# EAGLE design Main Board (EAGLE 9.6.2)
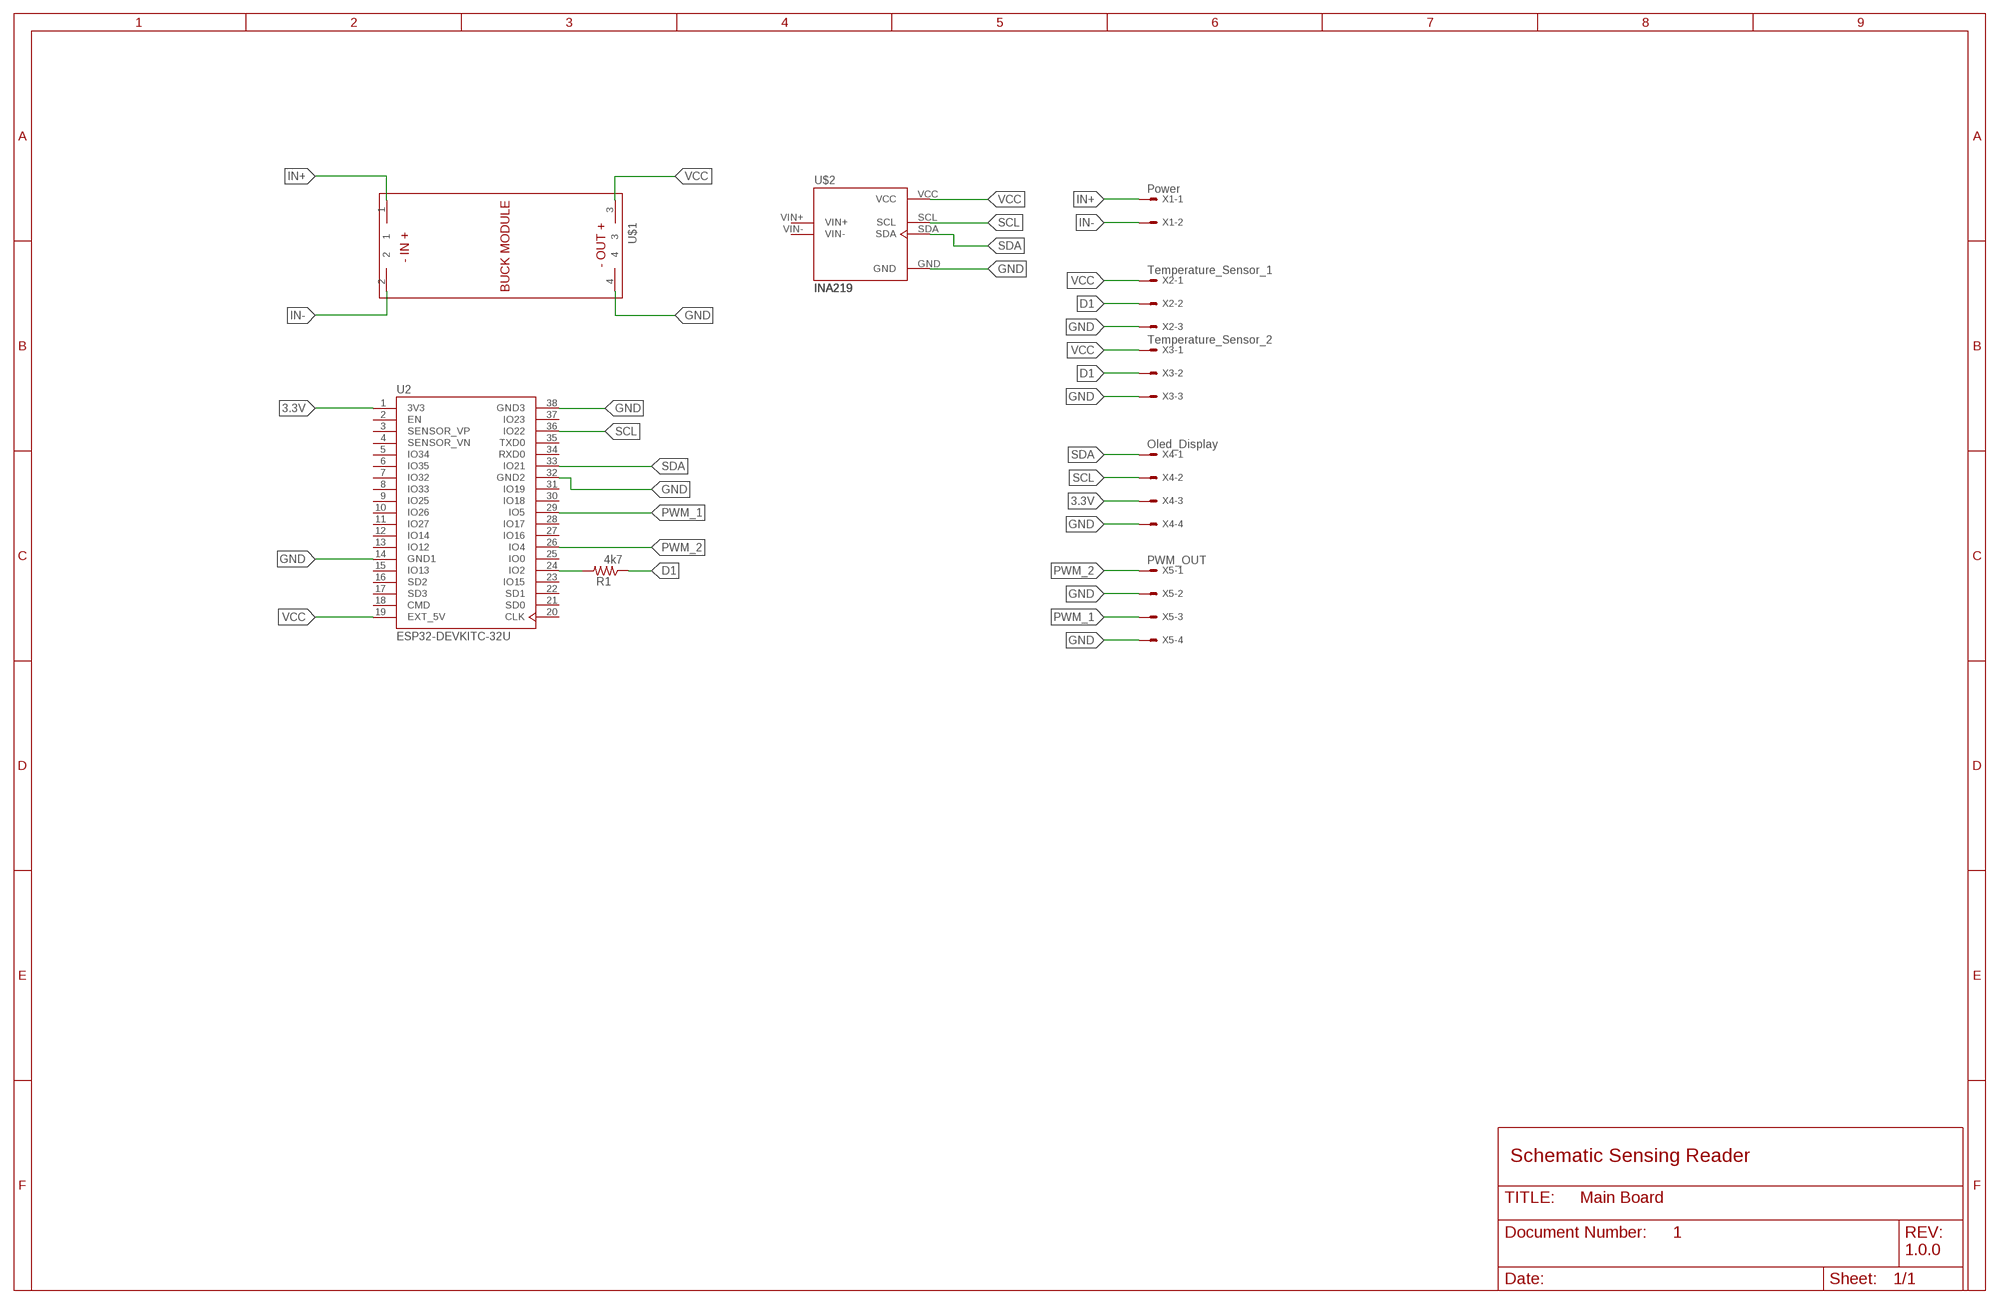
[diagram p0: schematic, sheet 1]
FRAME1 (FRAME_B_L): DESIGNER: PRATIK MAKWANA; DOC: 1; REV: 1.0.0

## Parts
R1  4k7  R-US_0207/10  [0207/10]
U2  ESP32-DEVKITC-32U  [MODULE_ESP32-DEVKITC-32U]
U$1  BUCK_MODULEWITH_SMDPADS&THROUGHHOLES  [BUCK_MODULE]
U$2  INA219  [INA219]
X1  Power  22-23-2021  [22-23-2021]
X2  Temperature_Sensor_1  22-23-2031  [22-23-2031]
X3  Temperature_Sensor_2  22-23-2031  [22-23-2031]
X4  Oled_Display  22-23-2041  [22-23-2041]
X5  PWM_OUT  22-23-2041  [22-23-2041]

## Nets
3.3V: U2.1(3V3) X4.3
D1: R1.1 X2.2 X3.2
GND: U2.14(GND1) U2.32(GND2) U2.38(GND3) U$1.4 U$2.GND X2.3 X3.3 X4.4 X5.2 X5.4
IN+: U$1.1 X1.1
IN-: U$1.2 X1.2
N$1: R1.2 U2.24(IO2)
PWM_1: U2.29(IO5) X5.3
PWM_2: U2.26(IO4) X5.1
SCL: U2.36(IO22) U$2.SCL X4.2
SDA: U2.33(IO21) U$2.SDA X4.1
VCC: U2.19(EXT_5V) U$1.3 U$2.VCC X2.1 X3.1
Unconnected: U2.2(EN) U2.3(SENSOR_VP) U2.4(SENSOR_VN) U2.5(IO34) U2.6(IO35) U2.7(IO32) U2.8(IO33) U2.9(IO25) U2.10(IO26) U2.11(IO27) U2.12(IO14) U2.13(IO12) U2.15(IO13) U2.16(SD2) U2.17(SD3) U2.18(CMD) U2.20(CLK) U2.21(SD0) U2.22(SD1) U2.23(IO15) U2.25(IO0) U2.27(IO16) U2.28(IO17) U2.30(IO18) U2.31(IO19) U2.34(RXD0) U2.35(TXD0) U2.37(IO23) U$2.VIN+ U$2.VIN-

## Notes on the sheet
- Schematic Sensing Reader

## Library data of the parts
R1 = adafruit:R-US_: RESISTOR, American symbol
U2 = ESP32-DEVKITC-32U:ESP32-DEVKITC-32U: Check availability; AVAILABILITY: In Stock; CHECK_PRICES: https://www.snapeda.com/parts/ESP32-DEVKITC-32U/Espressif+Systems/view-part/?ref=eda; DESCRIPTION: ESP32-WROOM-32UE series Transceiver; 802.11 b/g/n (Wi-Fi, WiFi, WLAN), Bluetooth® Smart Ready 4.x Dual Mode Evaluation Board; MF: Espressif Systems; MP: ESP32-DEVKITC-32U; PACKAGE: CUSTOM-38 ESPRESSIF; PRICE: None; SNAPEDA_LINK: https://www.snapeda.com/parts/ESP32-DEVKITC-32U/Espressif+Systems/view-part/?ref=snap
U$1 = BUCK_MODULE:BUCK_MODULE
U$2 = INA219:INA219
X1 = con-molex:22-23-2021: .100" (2.54mm) Center Header - 2 Pin; MF: MOLEX; MPN: 22-23-2021; OC_FARNELL: 1462926; OC_NEWARK: 25C3832
X2 X3 = con-molex:22-23-2031: .100" (2.54mm) Center Header - 3 Pin; MF: MOLEX; MPN: 22-23-2031; OC_FARNELL: 1462950; OC_NEWARK: 30C0862
X4 X5 = con-molex:22-23-2041: .100" (2.54mm) Center Header - 4 Pin; MF: MOLEX; MPN: 22-23-2041; OC_FARNELL: 1462920; OC_NEWARK: 38C0355

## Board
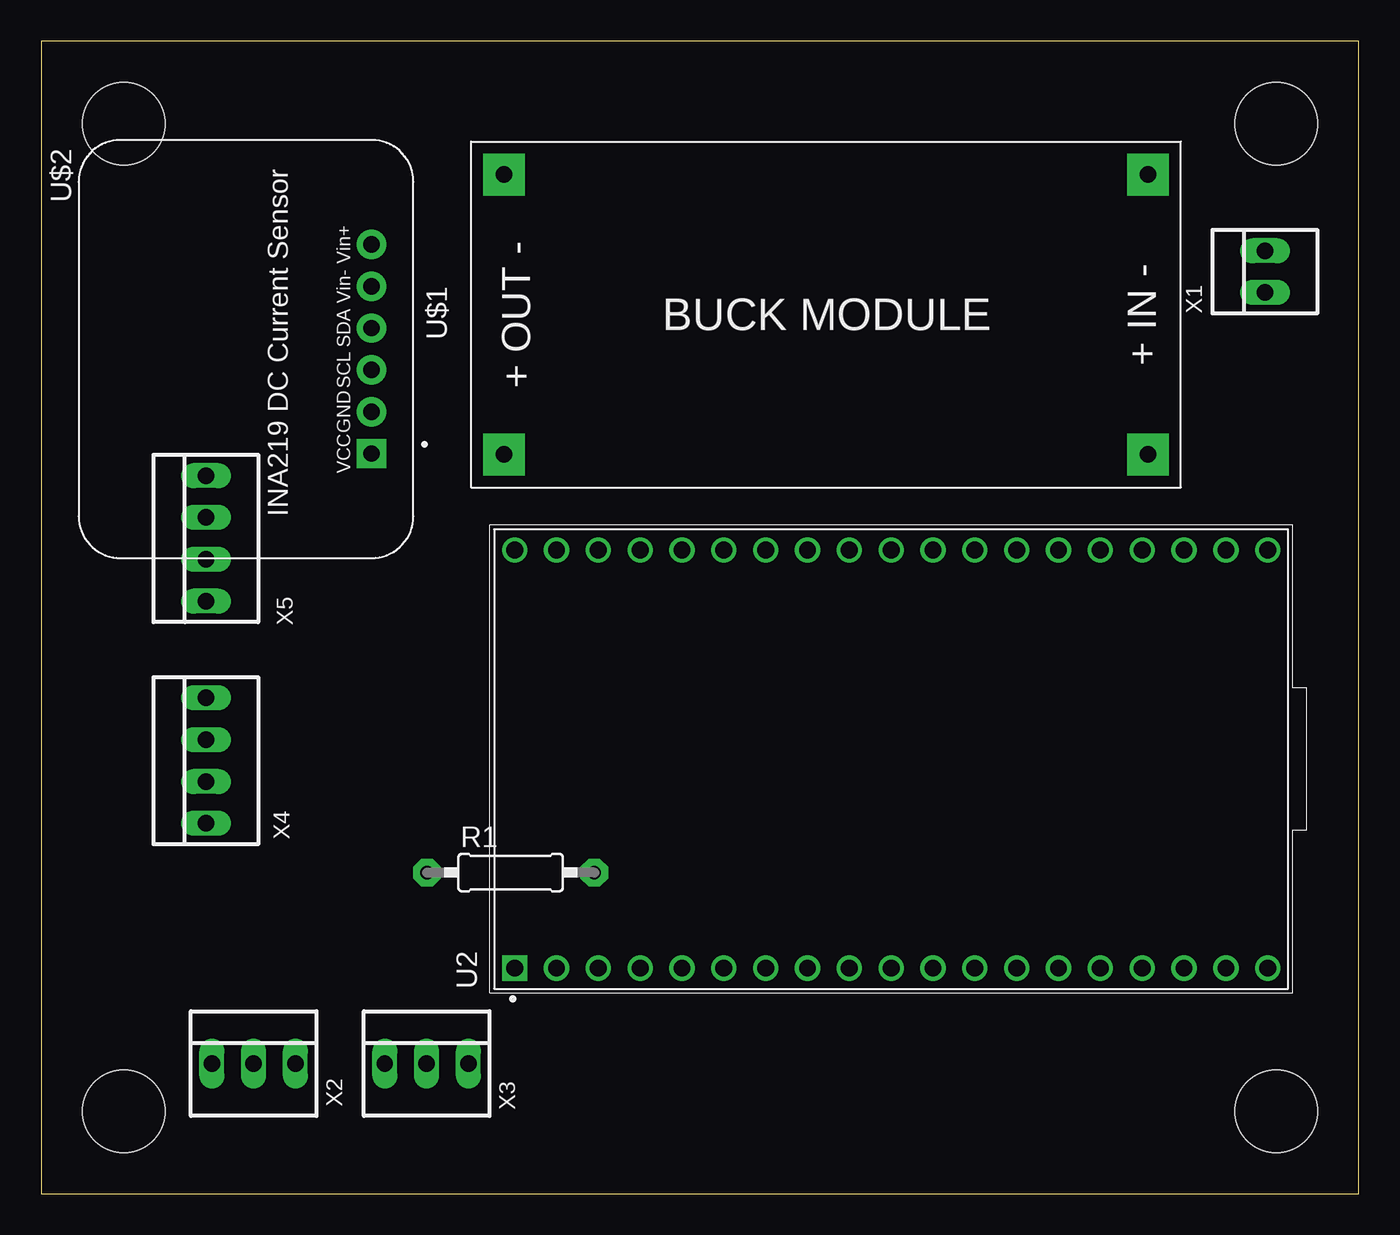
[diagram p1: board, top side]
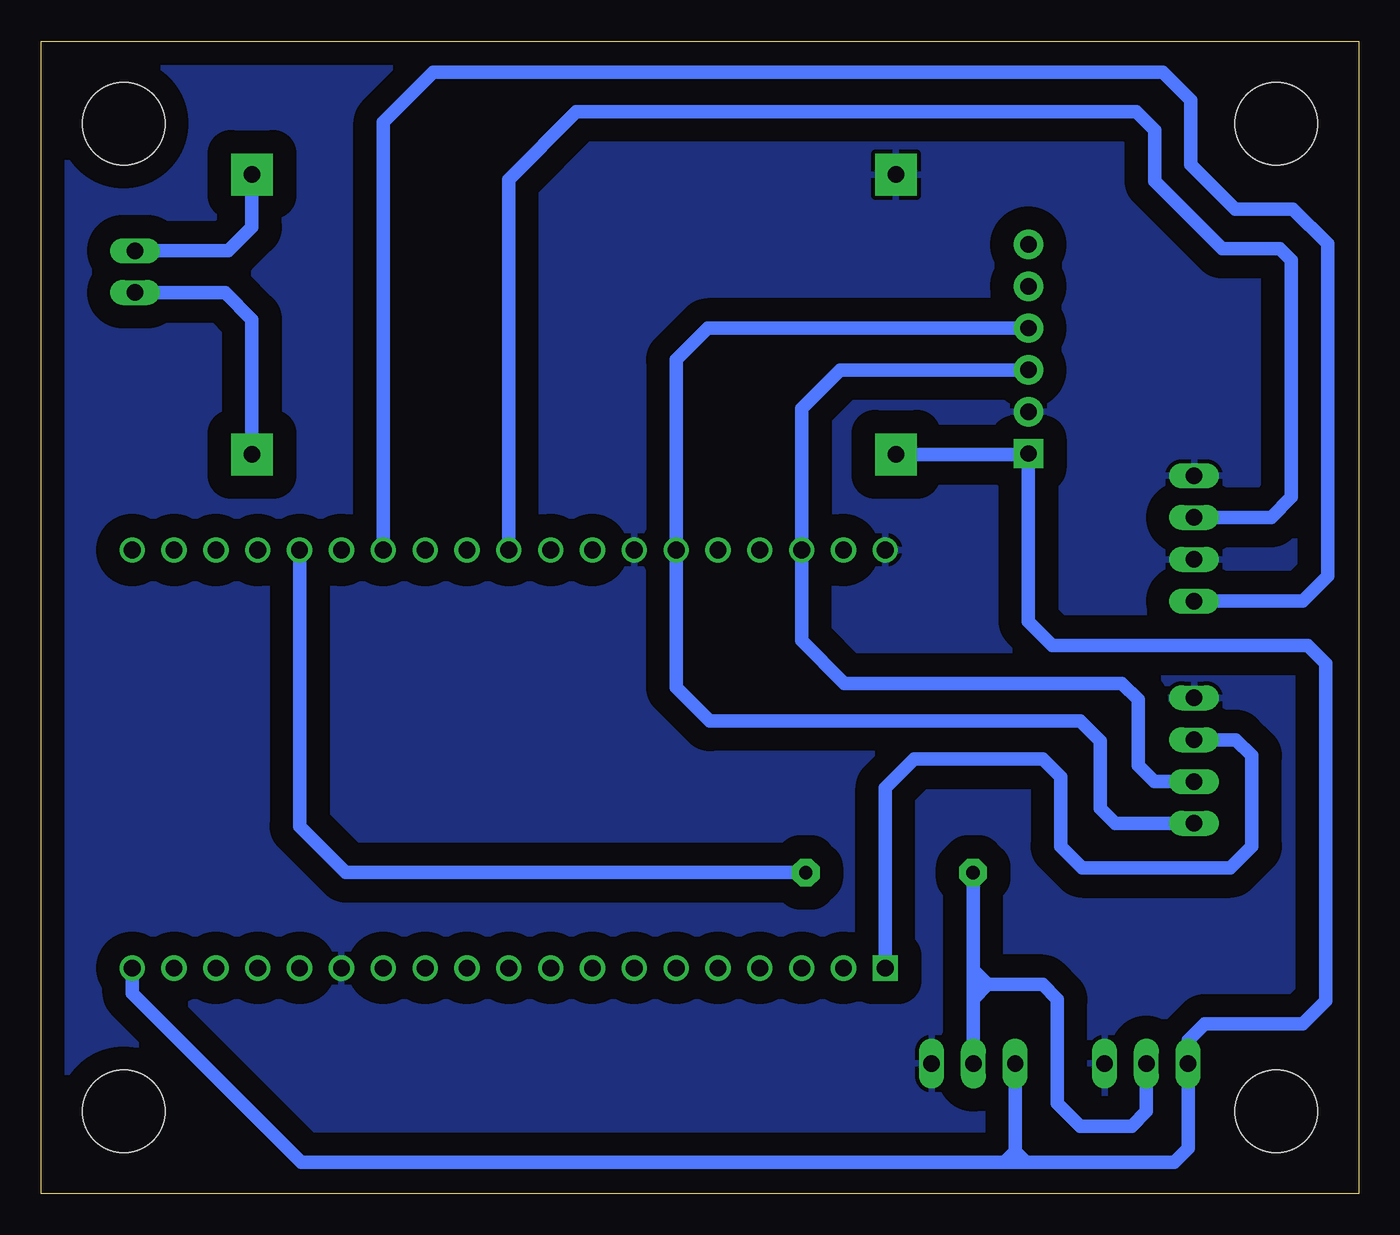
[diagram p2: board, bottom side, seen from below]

Size 80 x 70 mm. Coordinates in mm from the lower left corner, seen from the top.
Outline: 0,0 80,0 80,70 0,70 0,0
Copper layers (1*16): Top 0.035mm / dielectric 1.5mm / Bottom 0.035mm
Design rules "default": minimum track width 6mil, minimum drill 0.35mm, track to track 6mil, track to pad 6mil, pad to pad 6mil, via to via 6mil, smd to smd 6mil, copper to edge 40mil, drill to drill 6mil, minimum pad ring 10mil, minimum via ring 8mil, stop-mask expansion 4mil, vias tented up to drill 0mil, thermal gap 10mil
Holes 5 mm at 5,65 5,5 75,5 75,65

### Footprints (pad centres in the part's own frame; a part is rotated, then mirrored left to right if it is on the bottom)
0207/10 = drill 0.813 pad 1.676 octagon: 1 -5.08,0; 2 5.08,0
MODULE_ESP32-DEVKITC-32U = drill 1.02 square: 1 -12.7,22.85 | drill 1.02: 2 -12.7,20.31; 3 -12.7,17.77; 4 -12.7,15.23; 5 -12.7,12.69; 6 -12.7,10.15; 7 -12.7,7.61; 8 -12.7,5.07; 9 -12.7,2.53; 10 -12.7,-0.01; 11 -12.7,-2.55; 12 -12.7,-5.09; 13 -12.7,-7.63; 14 -12.7,-10.17; 15 -12.7,-12.71; 16 -12.7,-15.25; 17 -12.7,-17.79; 18 -12.7,-20.33; 19 -12.7,-22.87; 20 12.7,-22.87; 21 12.7,-20.33; 22 12.7,-17.79; 23 12.7,-15.25; 24 12.7,-12.71; 25 12.7,-10.17; 26 12.7,-7.63; 27 12.7,-5.09; 28 12.7,-2.55; 29 12.7,-0.01; 30 12.7,2.53; 31 12.7,5.07; 32 12.7,7.61; 33 12.7,10.15; 34 12.7,12.69; 35 12.7,15.23; 36 12.7,17.77; 37 12.7,20.31; 38 12.7,22.85
BUCK_MODULE = drill 1 pad 2.54 square: 1 -8.5,-19.5; 2 8.5,-19.5; 3 -8.5,19.6; 4 8.5,19.6
INA219 = drill 1 pad 1.778: GND 8.89,2.54; SCL 11.43,2.54; SDA 13.97,2.54; VIN+ 19.05,2.54; VIN- 16.51,2.54 | drill 1 pad 1.778 square: VCC 6.35,2.54
22-23-2021 = drill 1 long: 1 -1.27,0; 2 1.27,0
22-23-2031 = drill 1 long: 1 -2.54,0; 2 0,0; 3 2.54,0
22-23-2041 = drill 1 long: 1 -3.81,0; 2 -1.27,0; 3 1.27,0; 4 3.81,0

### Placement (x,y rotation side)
R1  28.5,19.5 0 top
U2  51.6,26.4 90 top
U$1  47.7,53.4 90 top
U$2  22.6,38.6 90 top
X1  74.3,56 90 top
X2  12.9,7.9 0 top
X3  23.4,7.9 0 top
X4  10,26.3 90 top
X5  10,39.8 90 top

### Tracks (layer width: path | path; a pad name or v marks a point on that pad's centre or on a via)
3.3V
  Bottom 0.813: X4.3 7.47,27.57 6.5,26.6 6.5,21.1 7.8,19.8 16.8,19.8 18.1,21.1 18.1,25.3 19.2,26.4 27,26.4 28.75,24.65 U2.1
D1
  Bottom 0.813: X2.2 12.9,5 13.8,4.1 16.9,4.1 18.3,5.5 18.3,11.8 19.2,12.7 22.52,12.7 | X3.2 23.42,7.92 23.42,11.8 | 23.42,11.8 23.42,13.6 | R1.1 23.42,14.1 23.42,13.6 | 22.52,12.7 23.42,11.8 | 22.52,12.7 23.42,13.6
GND
  pour Bottom (isolate 1.422): 0.2,69.9 79.9,69.9 79.9,0 0.2,0
IN+
  Bottom 0.813: X1.1 68.83,54.73 67.2,53.1 U$1.1
IN-
  Bottom 0.813: X1.2 68.63,57.27 67.2,58.7 U$1.2
N$1
  Bottom 0.813: R1.2 61.5,19.5 64.31,22.31 U2.24
PWM_1
  Bottom 0.813: U2.29 51.61,61.59 47.5,65.7 13.5,65.7 12.4,64.6 12.4,61.5 8.3,57.4 4.8,57.4 4.1,56.7 4.1,42.3 5.33,41.07 X5.3
PWM_2
  Bottom 0.813: U2.26 59.23,65.07 56.2,68.1 11.9,68.1 10.2,66.4 10.2,62.5 7.5,59.8 4,59.8 1.9,57.7 1.9,37.5 3.41,35.99 X5.1
SCL
  Bottom 0.813: U$2.SCL 31.47,50.03 33.83,47.67 U2.36 33.83,33.6 31.23,31 14.4,31 13.4,30 13.4,26 12.43,25.03 X4.2
SDA
  Bottom 0.813: U$2.SDA 39.53,52.57 41.45,50.65 U2.33 41.45,30.75 39.4,28.7 16.9,28.7 15.7,27.5 15.7,23.4 14.79,22.49 X4.1
VCC
  Bottom 0.813: U$1.3 20.11,44.9 U$2.VCC 20.06,34.76 18.6,33.3 3.1,33.3 2,32.2 2,11.7 3.4,10.3 9.36,10.3 10.36,9.3 X2.1 10.36,2.74 11.2,1.9 20.2,1.9 | 21.52,1.9 64.2,1.9 74.47,12.17 U2.19 | 21.52,1.9 20.2,1.9 | X3.1 20.86,2.56 | 20.2,1.9 20.86,2.56 | 20.86,2.56 21.52,1.9

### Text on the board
tValues: IN- | IN+ | GND | PWM_1 | GND | PWM_2 | GND | 3.3V | SCL | SDA | VCC | DATA | GND | VCC | DATA | GND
